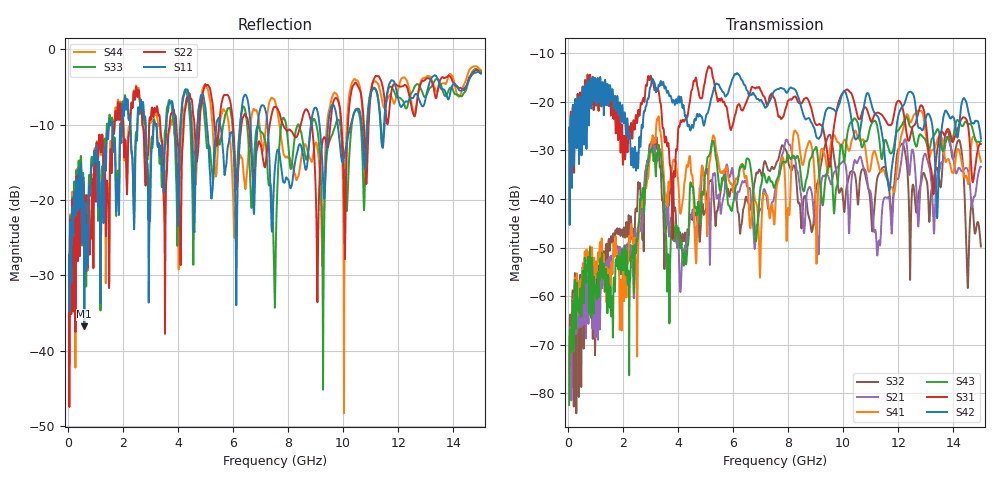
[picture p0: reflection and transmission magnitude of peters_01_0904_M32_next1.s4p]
# MHZ S RI R 50.00
! FREQ  S11  S12  S13  S14
!  S21  S22  S23  S24
!  S31  S32  S33  S34
!  S41  S42  S43  S44
!  REAL  IMAG  REAL  IMAG  REAL  IMAG  REAL  IMAG
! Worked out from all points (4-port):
!   1496 points, 50 MHz to 15 GHz, reference 50 ohm
!   strongest paths, dB at 50 MHz, 3.79 GHz, 7.53 GHz, 11.27 GHz, 15 GHz:
!     S42: -25.4, -20.0, -17.7, -23.2, -27.6
!     S31: -25.3, -41.6, -19.8, -22.2, -28.7
!     S43: -82.4, -40.9, -37.1, -26.1, -28.1
!     S41: -74.6, -33.2, -42.7, -32.6, -32.3
!     S21: -78.0, -44.7, -38.2, -49.6, -33.4
!     S32: -78.1, -35.0, -33.3, -35.2, -49.8
!   lowest |S11| = -36.8 dB at 600 MHz (marker M1), VSWR 1.03, Z = 49.5 - j1.37 ohm
!   |S11| at or under -10 dB: start of sweep to 1.496 GHz; 5.532 GHz to 6.265 GHz (733.9 MHz wide, 12.4 % of centre); 7.252 GHz to 8.83 GHz (1.578 GHz wide, 19.6 % of centre)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
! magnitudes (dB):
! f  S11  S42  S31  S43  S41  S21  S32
! 50 MHz  -27.3  -25.4  -25.3  -82.4  -74.6  -78.0  -78.1
! 600 MHz  -36.8  -27.1  -19.4  -56.1  -52.9  -56.6  -58.7
! 2.52 GHz  -11.6  -30.5  -24.4  -48.7  -72.4  -49.8  -42.1
! 3.09 GHz  -12.3  -15.4  -16.1  -30.0  -27.0  -29.0  -29.1
! 4.1 GHz  -10.3  -19.2  -23.9  -48.9  -43.0  -58.8  -48.9
! 13.78 GHz  -6.4  -22.2  -25.6  -27.5  -31.9  -27.2  -26.1
! 15 GHz  -3.3  -27.6  -28.7  -28.1  -32.3  -33.4  -49.8
